FUNCTION_BLOCK FB_LN_IED_LD1_LEDGGIO3 EXTENDS FB_AcsiCommonLogicalNodeClass
VAR_INPUT
	NamPlt: FB_DO_IED_LD1_LEDGGIO3_NamPlt := (sClass:='LPL', bLinkResult:=THIS^.AddDataToContainer(ipData:=NamPlt));
	Beh: FB_DO_IED_LD1_LEDGGIO3_Beh := (sClass:='ENS', bLinkResult:=THIS^.AddDataToContainer(ipData:=Beh));
	Health: FB_DO_IED_LD1_LEDGGIO3_Health := (sClass:='ENS', bLinkResult:=THIS^.AddDataToContainer(ipData:=Health));
	Mod_: FB_DO_IED_LD1_LEDGGIO3_Mod := (sObjectName:='Mod', sClass:='ENC', bLinkResult:=THIS^.AddDataToContainer(ipData:=Mod_));
	AnOut1: FB_DO_IED_LD1_LEDGGIO3_AnOut1 := (sClass:='APC', bLinkResult:=THIS^.AddDataToContainer(ipData:=AnOut1));
	SPCSO1: FB_DO_IED_LD1_LEDGGIO3_SPCSO1 := (sClass:='SPC', bLinkResult:=THIS^.AddDataToContainer(ipData:=SPCSO1));
	DPCSO1: FB_DO_IED_LD1_LEDGGIO3_DPCSO1 := (sClass:='DPC', bLinkResult:=THIS^.AddDataToContainer(ipData:=DPCSO1));
	ISCSO1: FB_DO_IED_LD1_LEDGGIO3_ISCSO1 := (sClass:='INC', bLinkResult:=THIS^.AddDataToContainer(ipData:=ISCSO1));
END_VAR
VAR
END_VAR

END_FUNCTION_BLOCK
